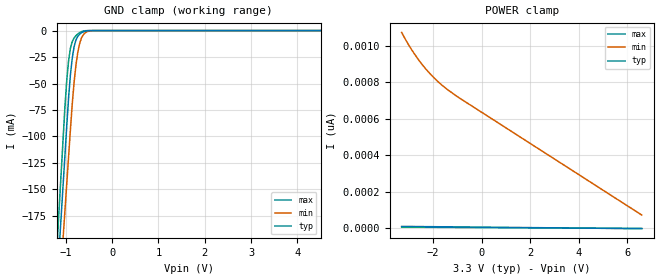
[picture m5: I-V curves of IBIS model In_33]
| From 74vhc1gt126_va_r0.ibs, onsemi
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|//////////////////////////////////////////////////////////////////////////////
|//////////////////////////////////////////////////////////////////////////////
[Model]  In_33
Model_type Input
Vinh = 1.40
Vinl = 0.45
|  variable   typ   min   max
C_comp   2.6pF   2.6pF   2.6pF
|//////////////////////////////////////////////////////////////////////////////
[Temperature Range]   25   125   -55
|//////////////////////////////////////////////////////////////////////////////
[Voltage Range]   3.30V   3.00V   3.60V
|//////////////////////////////////////////////////////////////////////////////
[POWER Clamp Reference] 3.30V   3.00V   3.60V
|//////////////////////////////////////////////////////////////////////////////
[GND Clamp Reference]   0V   0V   0V
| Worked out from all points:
|   GND clamp passes 1 mA (typ) near -0.61 V on its own axis
|//////////////////////////////////////////////////////////////////////////////
[GND Clamp]
|   Voltage   I(typ)   I(min)   I(max)
-3.3V     -1.731A    -1.647A    -1.822A
-1.24V    -274.5mA   -313.5mA   -241.9mA
-1.16V    -218mA     -261.7mA   -180.5mA
-1.1V     -175.5mA   -222.9mA   -134.5mA
-1.02V    -119mA     -171.1mA   -73.15mA
-940mV    -63.6mA    -119.3mA   -28.47mA
-860mV    -25.75mA   -68.96mA   -10.32mA
-780mV    -8.798mA   -32.28mA   -4.811mA
-740mV    -5.367mA   -20.28mA   -3.158mA
-660mV    -2.04mA    -6.802mA   -966.1uA
-380mV    -1.005uA   -28.62uA   -23.79nA
6.6V      8.236pA    943.7pA    4.015pA
|//////////////////////////////////////////////////////////////////////////////
[POWER Clamp]
|   Voltage   I(typ)   I(min)   I(max)
-3.3V     8.236pA    1.075nA    4.238pA
-2.92V    7.762pA    986.6pA    3.955pA
-2.44V    7.164pA    895.6pA    3.598pA
-1.92V    6.515pA    819.3pA    3.211pA
-1.44V    5.917pA    763.7pA    2.854pA
-960mV    5.318pA    717.8pA    2.497pA
6.6V      -4.109pA   70.82pA    -3.129pA
